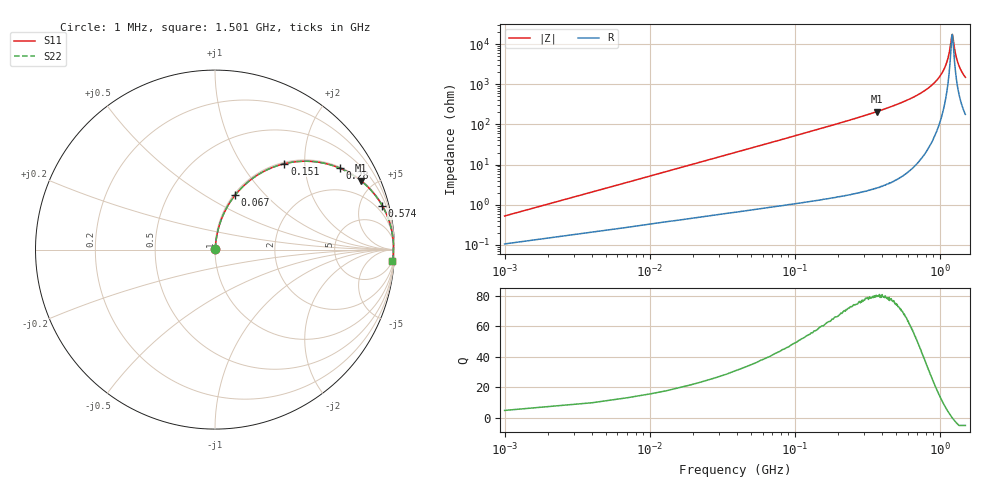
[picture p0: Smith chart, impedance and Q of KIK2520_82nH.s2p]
!version-2
!date-01.2022
!Series
# MHz S RI R 50
!Freq ReS11 ImS11 ReS21 ImS21 ReS12 ImS12 ReS22 ImS22
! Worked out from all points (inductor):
!   501 points, 1 MHz to 1.501 GHz, reference 50 ohm
!   read as one part in series: L = 82 nH near 7 MHz
!   highest Q = 79.9 at 370 MHz (marker M1), where L = 90.3 nH
!   self-resonance near 1.216 GHz
!   S11 on the Smith chart (normalised r, x): 1 MHz: 1.00, +0.01; 67 MHz: 1.02, +0.69; 151 MHz: 1.03, +1.58; 280 MHz: 1.04, +3.05; 574 MHz: 1.11, +7.60; 1.501 GHz: 5, -30
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1  0.00107 0.00514  0.9989 -0.00514  0.9989 -0.00514  0.00107 0.00514
10  0.00592 0.051  0.9941 -0.051  0.9941 -0.051  0.00592 0.051
19  0.0139 0.0961  0.9861 -0.0961  0.9861 -0.0961  0.0139 0.0961
37  0.0408 0.1819  0.9592 -0.1819  0.9592 -0.1819  0.0408 0.1819
67  0.1131 0.3045  0.8869 -0.3045  0.8869 -0.3045  0.1131 0.3045
103  0.2268 0.4088  0.7732 -0.4088  0.7732 -0.4088  0.2268 0.4088
151  0.3863 0.4786  0.6137 -0.4786  0.6137 -0.4786  0.3863 0.4786
253  0.6479 0.4709  0.3521 -0.4709  0.3521 -0.4709  0.6479 0.4709
280  0.6964 0.4533  0.3036 -0.4533  0.3036 -0.4533  0.6964 0.4533
370  0.8121 0.3844  0.1879 -0.3844  0.1879 -0.3844  0.8121 0.3844
502  0.9034 0.2887  0.0966 -0.2887  0.0966 -0.2887  0.9034 0.2887
574  0.9321 0.2443  0.0679 -0.2443  0.0679 -0.2443  0.9321 0.2443
751  0.9715 0.1551  0.0285 -0.1551  0.0285 -0.1551  0.9715 0.1551
1003  0.9917 0.0617  0.00832 -0.0617  0.00832 -0.0617  0.9917 0.0617
1129  0.9943 0.0242  0.00573 -0.0242  0.00573 -0.0242  0.9943 0.0242
1168  0.9944 0.0134  0.00557 -0.0134  0.00557 -0.0134  0.9944 0.0134
1213  0.9943 0.00154  0.00568 -0.00154  0.00568 -0.00154  0.9943 0.00154
1228  0.9942 -0.00232  0.00578 0.00232  0.00578 0.00232  0.9942 -0.00232
1252  0.994 -0.00841  0.00601 0.00841  0.00601 0.00841  0.994 -0.00841
1291  0.9935 -0.018  0.00655 0.018  0.00655 0.018  0.9935 -0.018
1342  0.9925 -0.0302  0.00752 0.0302  0.00752 0.0302  0.9925 -0.0302
1501  0.9878 -0.0651  0.0122 0.0651  0.0122 0.0651  0.9878 -0.0651
